ORGANIZATION_BLOCK MAIN:OB1
TITLE= Avviatore Stella-Triangolo per M.A.T.
// Simulatore: 02
// Versione: 1.0
// Data: 26/02/2002
//
//----------- Descrizione dell'impianto -----------------
// Il pulsante NA SB1 inserisce il contattore KM2
// predisposto per il collegamento a Stella del Motore e nello
// stesso tempo fa partire il temporizzatore T32 ritardato
// all'eccitazione.
// Il contatto NA di KM2 (KM2a) da il consenso all'eccitazione
// del contattore principale di linea KM1 e il motore funziona
// quindi a stella.
// Trascorso il tempo di ritardo (5 s) il contatto del temporizzatore
// T32 disinserisce il contattore di stella KM2.
// La disinserzione di KM2 da il consenso all'eccitazione del
// contattore KM3 e il motore marcia regolarmente a triangolo.
// Il pulsante NC SB1  può arrestare in qualsiasi momento
// la marcia del motore.
// I contattori KM3 e KM2 non possono essere inseriti conteporaneamente
// e quindi è necessario creare un interblocco elettrico hardware oltre
// a quello software gestito dal PLC.
// Il motore è protetto da un Relè termico FR.
// Per motivi di sicurezza il un contatto NC del Relè Termico
// FR viene collegato a monte della bobina dei contattori.
// Se inteviene la protezione le bobine dei contatori vengono
// disinserita direttamente via hardware senza l'intervento
// del controllore programmabile.
// Un contatto NC di RT viene però riportato anche su un
// ingresso  del PLC per disattivare le uscite in caso di
// intervento dello stesso e segnalare mediante la lampada
// HL1 il suo intervento.
// Le segnalazioni sono affidate a tre lampade che segnalano:
// HL2: lo stato di motore Fermo
// HL3: Lo Stato di motore in marcia a triangolo quando è
//      accesa in continuità e lo stato di marcia a stella
//      quando lampeggia.
// HL1: L'intervento del relè termico.

BEGIN
NETWORK 1 //Merker attivazione teleruttore stella
//
LD I0.1
AN Q0.0
LD Q0.0
A Q0.1
OLD
A I0.5
A I0.0
AN Q0.2
= M0.0

NETWORK 2 //Attivazione Contattore Stella
//
LD I0.5
A M0.0
AN T32
= Q0.1

NETWORK 3 //Temporizzatore Stella
//
LD M0.0
TON T32 +50

NETWORK 4 //Gestione Contattore di Linea
//
LD I0.1
A I0.4
O Q0.0
A I0.0
A I0.5
= Q0.0

NETWORK 5 //Gestione Contattore Triangolo
//
LD Q0.0
AN I0.4
= Q0.2

NETWORK 6 //Segnalazione Motore Fermo
//
LDN Q0.0
= Q0.3

NETWORK 7 //Segnalazione Marcia motore (Lampeggio a stella)
//
LD Q0.0
A Q0.2
LD SM0.5
A Q0.1
OLD
= Q0.4

NETWORK 8 //Segnalazione intervento relè termico
//
LDN I0.5
= Q0.6

END_ORGANIZATION_BLOCK

